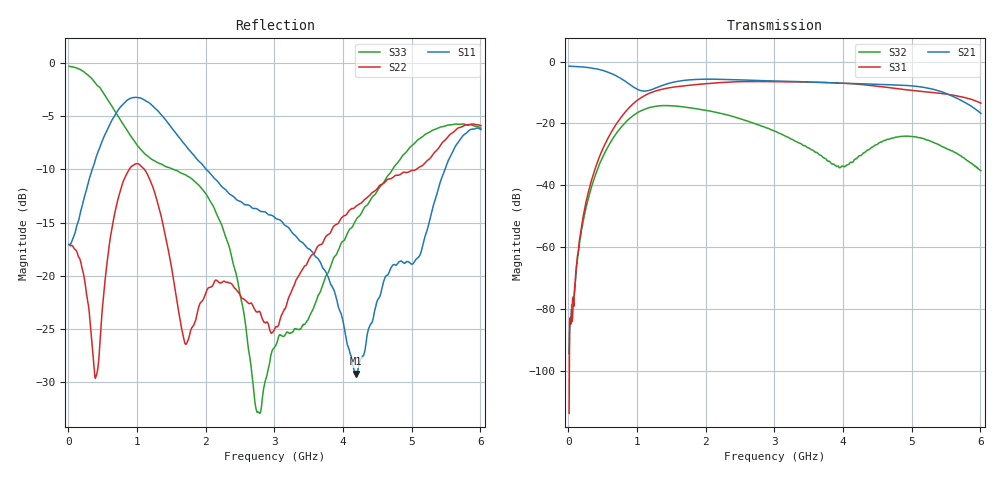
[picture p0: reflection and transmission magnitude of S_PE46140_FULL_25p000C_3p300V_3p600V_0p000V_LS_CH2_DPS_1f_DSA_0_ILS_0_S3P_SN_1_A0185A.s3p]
! Device ID: PE46140_FULL
! File Path: z:\PE46140\MajorStates\25p000C\3p300\LS_CH2_DPS_1f_DSA_0_ILS_0\PE46140_FULL_25p000C_3p300V_3p600V_0p000V_LS_CH2_DPS_1f_DSA_0_ILS_0_S3P_SN_1_A0185A.s3p
! Serial: 1
! Lot: A0185A
! Temp: 25.000C
! VDD: 3.300
! VSS: 0.000
! Control_Hi: 3.600
! Control_Lo: 0.000
! Logic State: LS_CH2_DPS_1f_DSA_0_ILS_0
! Port 1: RFIN
! Port 2: RFOUT1
! Port 3: RFOUT2
! ThroughPath:1-3
! IDD: 0.0003147101
! ISS: -2.242e-007
! Comment:
#  Hz  S  RI  R  50
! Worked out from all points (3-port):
!   801 points, 10 MHz to 6.01 GHz, reference 50 ohm
!   strongest paths, dB at 10 MHz, 1.51 GHz, 3.01 GHz, 4.51 GHz, 6.01 GHz:
!     S21: -1.5, -6.8, -6.3, -7.4, -16.8
!     S31: -113.8, -8.3, -6.5, -8.0, -13.5
!     S32: -94.6, -14.3, -22.6, -26.6, -35.3
!   lowest |S11| = -29.2 dB at 4.195 GHz (marker M1), VSWR 1.07, Z = 47.1 + j1.74 ohm
!   |S11| at or under -10 dB: start of sweep to 346.2 MHz; 2.008 GHz to 5.487 GHz (3.479 GHz wide, 92.8 % of centre)
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1e7  0.1401 -0.0109  0.8422 -0.0244  -5.92e-05 1.6e-06
     0.8417 -0.0244  0.1401 -0.00676  1.23e-05 -2.62e-05
     7.51e-07 -1.89e-06  1.32e-05 -1.32e-05  0.9668 -0.0408
3.475e8  -0.00846 -0.3171  0.4735 -0.6215  -0.0131 -0.00177
         0.4733 -0.6199  -0.00476 -0.0466  -0.00931 0.00452
         -0.0132 -0.00183  -0.00925 0.00446  0.2367 -0.8063
8.95e8  -0.6601 -0.1669  -0.2445 -0.3471  0.0338 0.1813
        -0.2439 -0.3477  0.3055 0.0949  0.1208 0.0101
        0.0334 0.1812  0.1207 0.0102  -0.4055 0.2187
1.375e9  -0.4483 0.3369  -0.3136 -0.2692  0.3431 -0.105
         -0.3135 -0.2695  0.0505 -0.1684  -0.1329 -0.1411
         0.3431 -0.1051  -0.133 -0.141  0.2647 0.2008
1.9375e9  -0.126 0.3133  -0.4707 0.2142  -0.0841 -0.4235
          -0.4708 0.2142  0.0723 -0.0215  -0.0236 0.1652
          -0.0844 -0.4235  -0.0236 0.1653  0.1721 -0.1921
2.755e9  -0.00245 0.2057  0.2353 0.4334  -0.4284 0.2042
         0.2348 0.4337  -0.0258 -0.0624  0.0445 -0.0845
         -0.4289 0.2042  0.0444 -0.0846  -0.021 0.00908
3.01e9  0.0119 0.1871  0.4063 0.2653  -0.2659 0.3897
        0.4061 0.2663  -0.0565 -0.000644  -0.0314 -0.0672
        -0.2665 0.39  -0.0315 -0.0674  0.0137 0.0445
4.195e9  -0.0294 0.0184  -0.1 -0.4277  0.4216 -0.0959
         -0.0992 -0.4282  0.1722 0.1254  -0.012 -0.0238
         0.4217 -0.0957  -0.0121 -0.024  0.1027 0.1526
5.2525e9  -0.044 -0.1705  -0.1632 0.331  -0.1999 -0.2502
          -0.1641 0.3307  0.3523 -0.0167  0.0523 0.00805
          -0.1992 -0.2507  0.0522 0.00799  0.4591 -0.1099
6.01e9  -0.4559 -0.1715  0.14 0.0381  -0.1764 0.1176
        0.14 0.0382  0.2479 -0.4441  -0.0134 -0.0104
        -0.1761 0.1182  -0.0136 -0.0106  0.1922 -0.4558
